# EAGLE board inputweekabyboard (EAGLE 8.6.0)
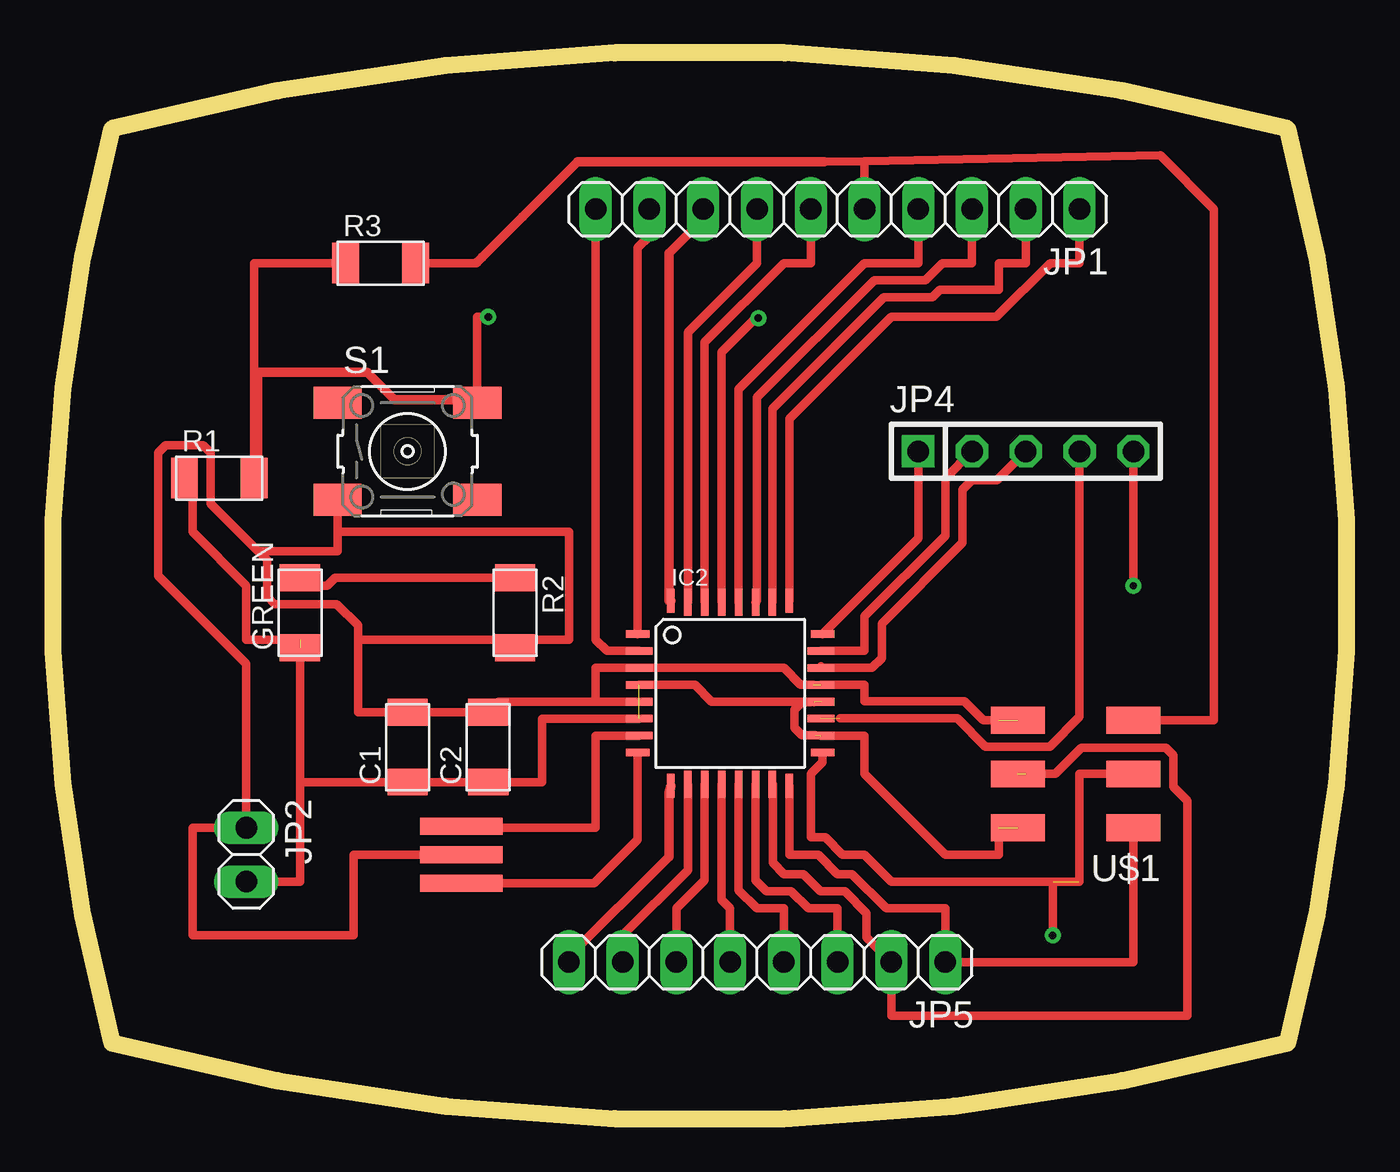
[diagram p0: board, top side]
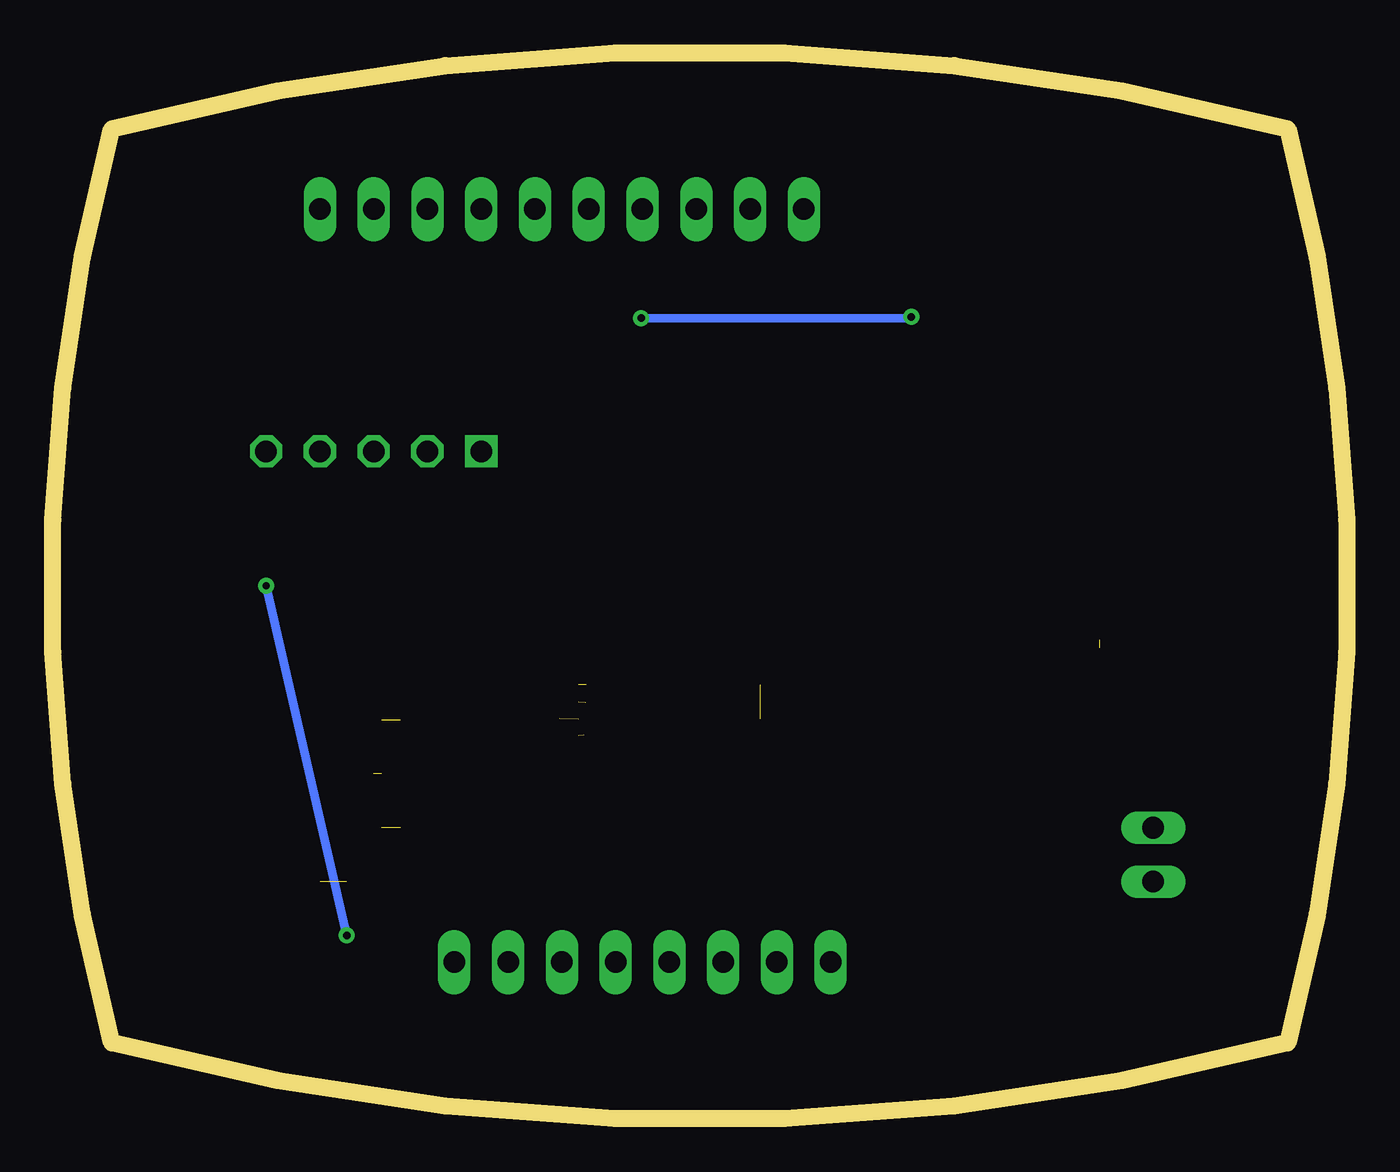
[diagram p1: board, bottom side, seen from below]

Size 61.12 x 50.33 mm. Coordinates in mm from the lower left corner, seen from the top.
Outline: 2.78,3.58 arc30 58.33,3.58 arc30 58.33,46.75 arc30 2.78,46.75 arc30 2.78,3.58
Copper layers (1*16): Top 0.035mm / dielectric 1.5mm / Bottom 0.035mm
Design rules "default *": minimum track width 18mil, minimum drill 0.35mm, track to track 16mil, track to pad 16mil, pad to pad 16mil, via to via 16mil, smd to smd 16mil, copper to edge 40mil, drill to drill 6mil, minimum pad ring 10mil, minimum via ring 8mil, stop-mask expansion 4mil, vias tented up to drill 0mil, thermal gap 10mil

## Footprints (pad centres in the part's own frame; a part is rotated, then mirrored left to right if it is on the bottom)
C1206FAB = smd 1.27 x 1.905: 1 -1.651,0; 2 1.651,0
LED1206FAB = smd 1.27 x 1.905: 1 -1.651,0; 2 1.651,0
TQFP32-08THIN = smd 1.118 x 0.356: 1 -4.369,2.8; 8 -4.369,-2.8; 17 4.369,-2.8; 24 4.369,2.8 | smd 1.27 x 0.356: 2 -4.293,2; 3 -4.293,1.2; 4 -4.293,0.4; 5 -4.293,-0.4; 6 -4.293,-1.2; 7 -4.293,-2; 18 4.293,-2; 19 4.293,-1.2; 20 4.293,-0.4; 21 4.293,0.4; 22 4.293,1.2; 23 4.293,2 | smd 0.356 x 1.118: 9 -2.8,-4.369; 16 2.8,-4.369; 25 2.8,4.369; 32 -2.8,4.369 | smd 0.356 x 1.27: 10 -2,-4.293; 14 1.2,-4.293; 15 2,-4.293; 26 2,4.293; 27 1.2,4.293; 31 -2,4.293 | smd 0.35 x 1.27: 11 -1.2,-4.293; 12 -0.4,-4.293; 13 0.4,-4.293; 28 0.4,4.293; 29 -0.4,4.293; 30 -1.2,4.293
1X10 = drill 1.016 long: 1 -11.43,0; 2 -8.89,0; 3 -6.35,0; 4 -3.81,0; 5 -1.27,0; 6 1.27,0; 7 3.81,0; 8 6.35,0; 9 8.89,0; 10 11.43,0
1X02 = drill 1.016 long: 1 -1.27,0; 2 1.27,0
1X05 = drill 1.016 square: 1 -5.08,0 | drill 1.016 octagon: 2 -2.54,0; 3 0,0; 4 2.54,0; 5 5.08,0
1X08 = drill 1.016 long: 1 -8.89,0; 2 -6.35,0; 3 -3.81,0; 4 -1.27,0; 5 1.27,0; 6 3.81,0; 7 6.35,0; 8 8.89,0
R1206FAB = smd 1.27 x 1.905: 1 -1.651,0; 2 1.651,0
6MM_SWITCH = smd 2.286 x 1.524: 1 -3.302,2.286; 2 3.302,2.286; 3 -3.302,-2.286; 4 3.302,-2.286
2X03SMD = smd 2.54 x 1.27: 1 -2.54,2.54; 2 2.92,2.54; 3 -2.54,0; 4 2.92,0; 5 -2.54,-2.54; 6 2.92,-2.54
EFOBM = smd 0.8 x 3.9: 1 -1.35,0; 2 0,0; 3 1.35,0

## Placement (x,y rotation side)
C1  1 uF  [C1206FAB]  16.75,17.55 90 top
C2  100 pF  [C1206FAB]  20.56,17.55 90 top
GREEN  LEDFAB1206  [LED1206FAB]  11.67,23.9 90 top
IC2  ATMEGA88-THIN  [TQFP32-08THIN]  31.99,20.09 0 top
JP1  [1X10]  37.07,42.95 180 top
JP2  [1X02]  9.13,12.47 270 top
JP4  [1X05]  45.96,31.52 0 top
JP5  [1X08]  33.26,7.39 180 top
R1  10 K  [R1206FAB]  7.86,30.25 0 top
R2  499 ohm  [R1206FAB]  21.83,23.9 270 top
R3  0 ohm  [R1206FAB]  15.48,40.41 0 top
S1  [6MM_SWITCH]  16.75,31.52 0 top
U$1  AVRISPSMD  [2X03SMD]  48.5,16.28 180 top
U$3  RESONATOR  [EFOBM]  19.29,12.47 270 top

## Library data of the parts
C1 C2 GREEN IC2 R1-R3 S1 U$1 U$3 = fab
JP1 JP2 JP4 JP5 = pinhead

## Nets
GND: C1.2 C2.2 IC2.3 IC2.5 IC2.21 JP2.1 R2.2 S1.3 U$1.6 U$3.2
N$1: IC2.7 U$3.1
N$2: IC2.8 U$3.3
N$3: IC2.29 R1.2 R3.1 S1.2
N$4: JP1.5 R3.2 U$1.5
N$5: IC2.17 JP4.5 U$1.3
N$6: IC2.16 JP5.1 U$1.1
N$7: IC2.15 JP5.2 U$1.4
N$8: GREEN.2 R2.1
N$9: IC2.19 JP4.4
N$10: IC2.22 JP4.3
N$11: IC2.23 JP4.2
N$12: IC2.24 JP4.1
N$13: IC2.9 JP5.8
N$14: IC2.2 JP1.10
N$15: IC2.1 JP1.9
N$16: IC2.32 JP1.8
N$17: IC2.31 JP1.7
N$18: IC2.30 JP1.6
N$19: IC2.28 JP1.4
N$20: IC2.27 JP1.3
N$21: IC2.26 JP1.2
N$22: IC2.25 JP1.1
N$23: IC2.10 JP5.7
N$24: IC2.11 JP5.6
N$25: IC2.12 JP5.5
N$26: IC2.13 JP5.4
N$27: IC2.14 JP5.3
VCC: C1.1 C2.1 GREEN.1 IC2.4 IC2.6 IC2.18 IC2.20 JP2.2 R1.1 U$1.2

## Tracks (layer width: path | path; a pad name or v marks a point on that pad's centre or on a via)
GND  (2 unrouted)
  Top 0.406: 14.42,22.63 14.42,23.31 13.41,24.31 10.47,24.31 10.11,24.66 10.11,26.39 9.71,26.8 | 14.42,22.63 14.42,19.2 C1.2 C2.2 21.05,19.69 25.64,19.69 | IC2.5 25.64,19.69 | U$3.2 14.21,12.47 14.21,8.66 6.59,8.66 6.59,13.74 JP2.1 9.13,21.48 7.92,22.69 4.97,25.65 4.97,31.46 5.32,31.81 7.1,31.81 7.46,31.46 7.46,29.05 9.71,26.8 | 25.64,19.69 25.64,21.29 IC2.3 34.53,21.29 35.32,20.5 35.92,20.5 | 9.71,26.8 13.45,26.8 13.45,27.71 | S1.3 13.45,27.71 | 14.42,22.63 21.45,22.63 R2.2 22.21,22.63 24.37,22.63 24.37,27.71 13.45,27.71 | IC2.21 38.34,20.49 38.34,19.72 43.07,19.72 43.97,18.82 44.69,18.82
  Top 0.457: 13.55,29.21 S1.3
N$1
  Top 0.406: IC2.7 25.64,18.09 25.64,13.74 19.29,13.74 U$3.1
N$2
  Top 0.406: IC2.8 27.62,13.18 25.56,11.12 U$3.3
N$3  (via drill 0.35)
  Top 0.406: IC2.29 31.59,36.2 33.26,37.87 v33.33,37.81 | v20.56,37.87 20.03,37.87 20.03,33.96 | R1.2 9.51,40.41 R3.1
  Top 0.457: R1.2 9.67,30.51 9.67,35.26 14.85,35.26 16.14,33.96 20.03,33.96 S1.2
  Bottom 0.406: v33.33,37.81 20.56,37.81 v20.56,37.87
N$4
  Top 0.406: 38.35,45.22 52.31,45.49 54.85,42.95 54.85,18.82 U$1.5 | 38.35,45.22 36.44,45.19 | JP1.5 38.35,45.22 | 20.28,40.69 20,40.41 R3.2
  Top 0.457: 20.03,40.44 20.28,40.69 22.19,42.6 24.78,45.19 36.44,45.19
N$5  (via drill 0.35)  (1 unrouted)
  Top 0.406: 51.04,16.71 U$1.3 48.5,16.28 48.5,11.2 39.61,11.2 38.34,12.47 37.31,12.47 36.5,13.28 35.8,13.28 35.8,16.28 36.36,16.84 IC2.17 | JP4.5 v51.04,25.17 | v47.23,8.66 47.23,11.2
  Bottom 0.406: v51.04,25.17 v47.23,8.66
N$6
  Top 0.406: IC2.16 34.79,12.47 36.16,12.47 37.07,11.56 37.75,11.56 39.37,9.93 42.15,9.93 JP5.1 51.04,7.39 U$1.1
N$7  (1 unrouted)
  Top 0.406: IC2.15 34.01,15.79 34.01,12.08 34.53,11.56 35.45,11.56 36.26,10.74 37.41,10.74 38.45,9.71 38.45,8.56 JP5.2 39.61,4.85 53.58,4.85 53.58,15.01 52.92,15.67 52.92,17.17 52.57,17.53 48.6,17.53 47.35,16.28 45.96,16.28 45.96,16.13
N$8
  Top 0.406: R2.1 13.32,25.55 12.94,25.17 12.05,25.17 GREEN.2
N$9  (1 unrouted)
  Top 0.406: 37.17,18.9 42.73,18.9 44.06,17.58 47.11,17.58 48.5,18.97 JP4.4
N$10
  Top 0.406: 36.29,21.36 IC2.22 38.69,21.29 39.16,21.75 39.16,23.39 42.97,27.2 42.97,29.69 43.42,30.15 44.59,30.15 JP4.3
N$11
  Top 0.406: JP4.2 42.15,30.25 42.15,27.53 38.34,23.72 38.34,22.09 IC2.23
N$12
  Top 0.406: IC2.24 40.88,27.41 JP4.1
N$13
  Top 0.457: IC2.9 29.1,15.39 29.1,12.37 24.35,7.62 JP5.8
N$14
  Top 0.406: IC2.2 26.18,22.09 25.64,22.63 JP1.10
N$15
  Top 0.406: IC2.1 27.62,41.12 28.18,41.68 JP1.9
N$16
  Top 0.457: IC2.32 29.1,24.46 29.1,40.87 30.83,42.6 JP1.8
N$17
  Top 0.406: IC2.31 29.99,37.14 33.26,40.41 JP1.7
N$18
  Top 0.406: IC2.30 30.79,36.67 34.53,40.41 35.8,40.41 JP1.6
N$19
  Top 0.406: IC2.28 32.39,34.46 38.34,40.41 40.88,40.41 JP1.4
N$20
  Top 0.406: IC2.27 33.26,24.45 33.26,34.06 38.8,39.6 41.22,39.6 42.03,40.41 43.42,40.41 JP1.3
N$21
  Top 0.406: IC2.26 33.99,33.52 39.26,38.79 41.56,38.79 41.91,39.14 44.69,39.14 44.69,40.41 45.96,40.41 JP1.2
N$22
  Top 0.406: IC2.25 34.79,33.05 39.61,37.87 44.57,37.87 47.11,40.41 48.5,40.41 JP1.1
N$23
  Top 0.406: IC2.10 29.99,11.74 26.91,8.66 JP5.7
N$24
  Top 0.406: IC2.11 30.79,11.27 29.45,9.93 JP5.6
N$25
  Top 0.406: IC2.12 31.59,10.33 31.99,9.93 JP5.5
N$26
  Top 0.406: IC2.13 32.39,10.8 33.26,9.93 34.53,9.93 JP5.4
N$27
  Top 0.406: IC2.14 33.19,11.27 33.72,10.74 34.87,10.74 35.68,9.93 37.07,9.93 JP5.3
VCC  (5 unrouted)
  Top 0.406: IC2.4 30.32,20.49 31.12,19.69 35.8,19.69 | 35.95,19.68 35.94,19.69 35.8,19.69 | 36.03,18.1 35.4,18.1 35.04,18.46 35.04,19.32 35.4,19.68 35.79,19.68 35.8,19.69 | IC2.6 23.1,18.89 23.1,15.9 C2.1 C1.1 11.67,15.9 | 11.67,15.9 11.67,11.2 JP2.2 | IC2.18 38.34,18.09 38.34,16.28 42.15,12.47 44.69,12.47 44.69,13.74 | GREEN.1 11.67,15.9 | R1.1 6.59,29.87 6.59,27.71 9.13,25.17 9.13,22.63 11.67,22.63
  Top 0.457: 6.21,30.07 R1.1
